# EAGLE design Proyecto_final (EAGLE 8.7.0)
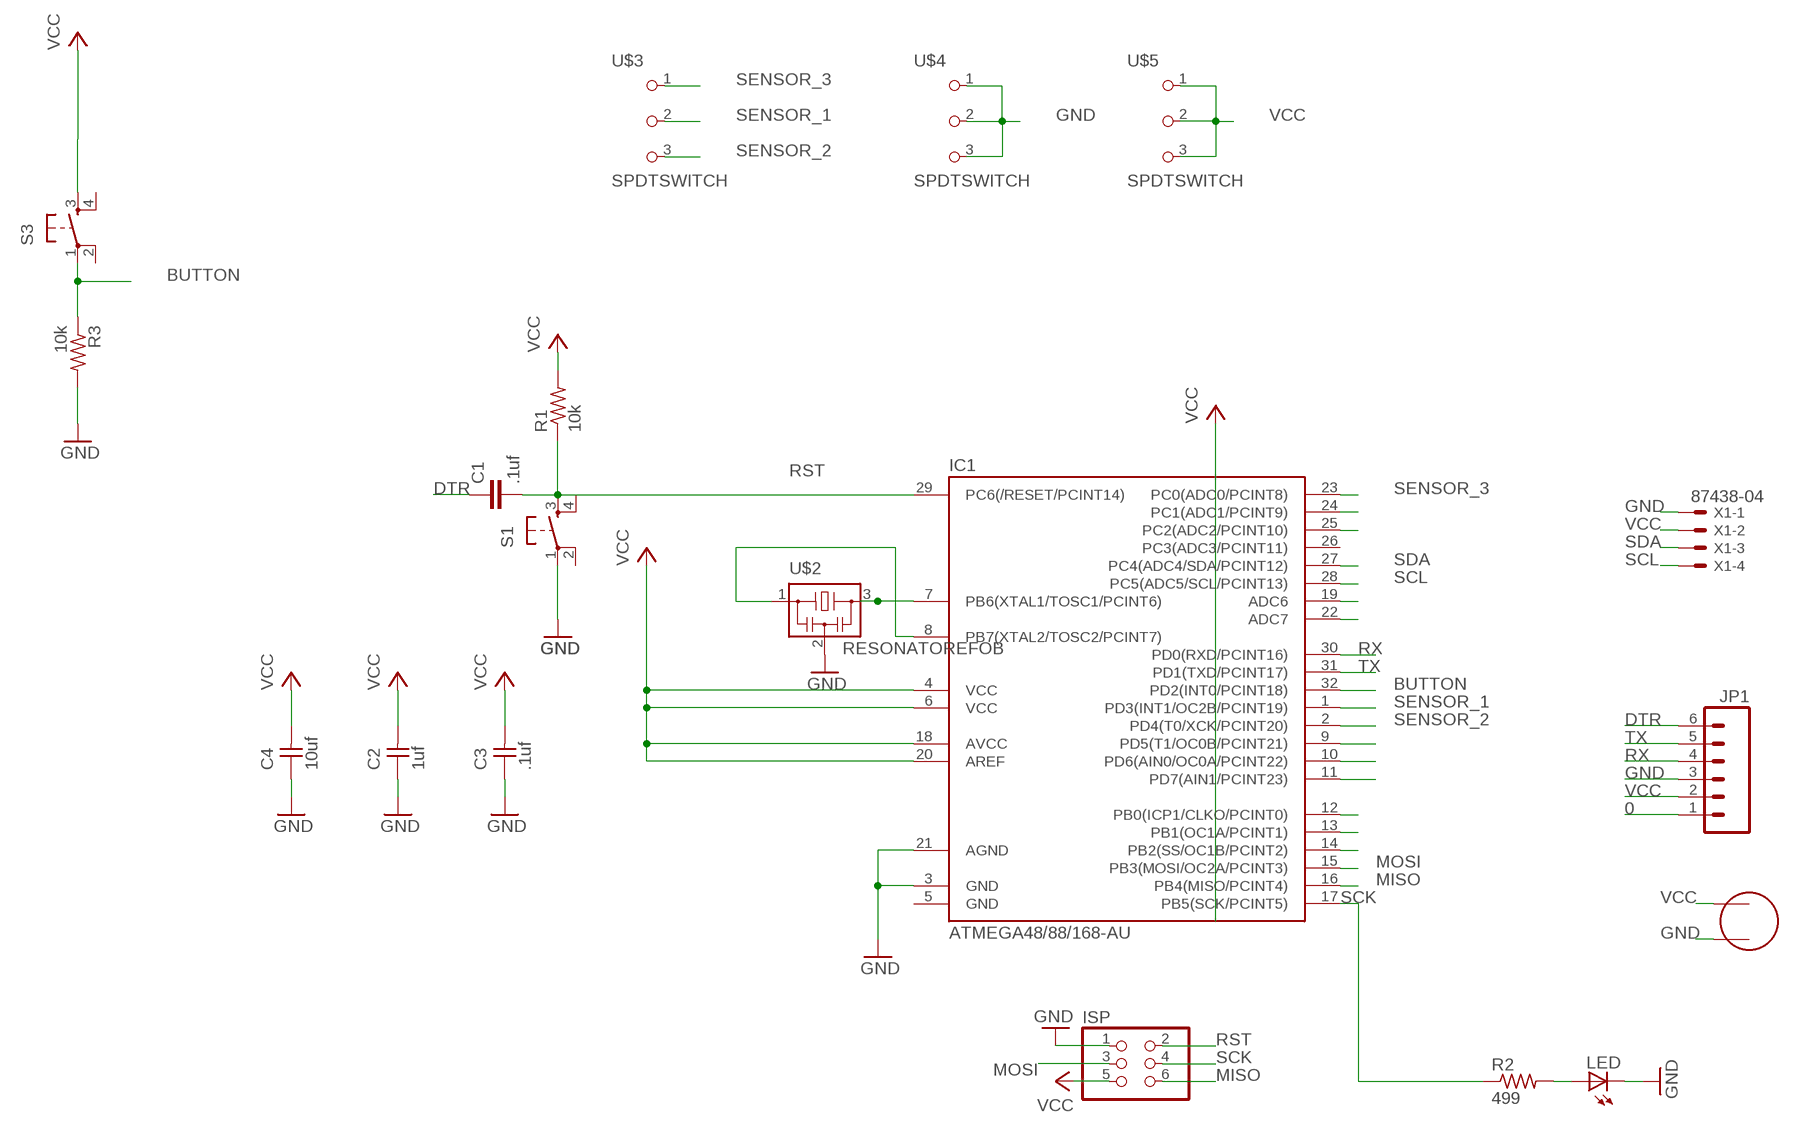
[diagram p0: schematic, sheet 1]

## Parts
C1  .1uf  C-EUC1206  [C1206]
C2  1uf  UNPOLARIZED_CAPACITOR1206  [1206]
C3  .1uf  UNPOLARIZED_CAPACITOR1206  [1206]
C4  10uf  UNPOLARIZED_CAPACITOR1206  [1206]
IC1  ATMEGA48/88/168-AU  [TQFP32-08]
ISP  PINHD-2X3-SMD  [2X03SMD]
JP1  M06SMD  [1X06-SMD]
LED  LED1206  [1206]
R1  10k  RESISTOR1206  [1206]
R2  499  RESISTOR1206  [1206]
R3  10k  RESISTOR1206  [1206]
S1  6MM_SWITCH6MM_SWITCH  [6MM_SWITCH]
S3  6MM_SWITCH6MM_SWITCH  [6MM_SWITCH]
U$1  ELECTRET  [ELECTRET_2742PBJ-A]
U$2  RESONATOREFOB  [EFOBM]
U$3  SPDTSWITCH  [SPDTSWITCH]
U$4  SPDTSWITCH  [SPDTSWITCH]
U$5  SPDTSWITCH  [SPDTSWITCH]
X1  87438-04  [87438-04]

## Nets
0: JP1.1
BUTTON: IC1.32(PD2(INT0/PCINT18)) R3.1 S3.1(P)
DTR: C1.1 JP1.6
GND: C2.1 C3.1 C4.1 IC1.3(GND) IC1.21(AGND) ISP.1 JP1.3 LED.2(C) R3.2 S1.1(P) U$1.P$2 U$2.2 U$4.1 U$4.2 U$4.3 X1.1
MISO: IC1.16(PB4(MISO/PCINT4)) ISP.6
MOSI: IC1.15(PB3(MOSI/OC2A/PCINT3)) ISP.3
N$1: IC1.8(PB7(XTAL2/TOSC2/PCINT7)) U$2.1
N$4: IC1.25(PC2(ADC2/PCINT10))
N$8: IC1.19(ADC6)
N$9: IC1.7(PB6(XTAL1/TOSC1/PCINT6)) U$2.3
N$10: IC1.22(ADC7)
N$14: IC1.9(PD5(T1/OC0B/PCINT21))
N$15: IC1.10(PD6(AIN0/OC0A/PCINT22))
N$16: IC1.11(PD7(AIN1/PCINT23))
N$17: IC1.14(PB2(SS/OC1B/PCINT2))
N$18: IC1.13(PB1(OC1A/PCINT1))
N$19: IC1.12(PB0(ICP1/CLKO/PCINT0))
N$23: LED.1(A) R2.2
RST: C1.2 IC1.29(PC6(/RESET/PCINT14)) ISP.2 R1.1 S1.3(S)
RST1: S3.3(S)
RX: IC1.30(PD0(RXD/PCINT16)) JP1.4
SCK: IC1.17(PB5(SCK/PCINT5)) ISP.4 R2.1
SCL: IC1.28(PC5(ADC5/SCL/PCINT13)) X1.4
SDA: IC1.27(PC4(ADC4/SDA/PCINT12)) X1.3
SENSOR_1: IC1.1(PD3(INT1/OC2B/PCINT19)) U$3.2
SENSOR_2: IC1.2(PD4(T0/XCK/PCINT20)) U$3.3
SENSOR_3: IC1.23(PC0(ADC0/PCINT8)) IC1.24(PC1(ADC1/PCINT9)) U$3.1
TX: IC1.31(PD1(TXD/PCINT17)) JP1.5
VCC: C2.2 C3.2 C4.2 IC1.4(VCC) IC1.6(VCC) IC1.18(AVCC) IC1.20(AREF) ISP.5 JP1.2 R1.2 U$1.P$1 U$5.1 U$5.2 U$5.3 X1.2
Unconnected: IC1.26(PC3(ADC3/PCINT11)) S1.2(P1) S1.4(S1) S3.2(P1) S3.4(S1)

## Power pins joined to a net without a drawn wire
GND: IC1.5(GND)

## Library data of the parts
C1 = rcl:C-EU: CAPACITOR, European symbol
C2-C4 = ng:UNPOLARIZED_CAPACITOR: unpolarized_capacitor
IC1 = atmega8:ATMEGA48/88/168
ISP = fab:PINHD-2X3-SMD: PIN HEADER
JP1 = SparkFun:M06: Header 6 Standard 6-pin 0.1" header. Use with straight break away headers (SKU : PRT-00116), right angle break away headers (PRT-00553), swiss pins (PRT-00743), machine pins (PRT-00117), and female headers (PRT-00115). Molex polarized connector foot print use with SKU : PRT-08094 with associated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
LED = ng:LED
R1-R3 = ng:RESISTOR
S1 S3 = ng:6MM_SWITCH: OMRON SWITCH
U$1 = fab:ELECTRET
U$2 = fab:RESONATOR
U$3-U$5 = fab:SPDTSWITCH
X1 = con-molex:87438-04: Wire-to-Board 1.50mm (.059") Pitch Header - Right Angle, SMT, Shrouded Source: http://www.molex.com/product/micro/87438.html; MF: MOLEX; OC_FARNELL: unknown; OC_NEWARK: unknown

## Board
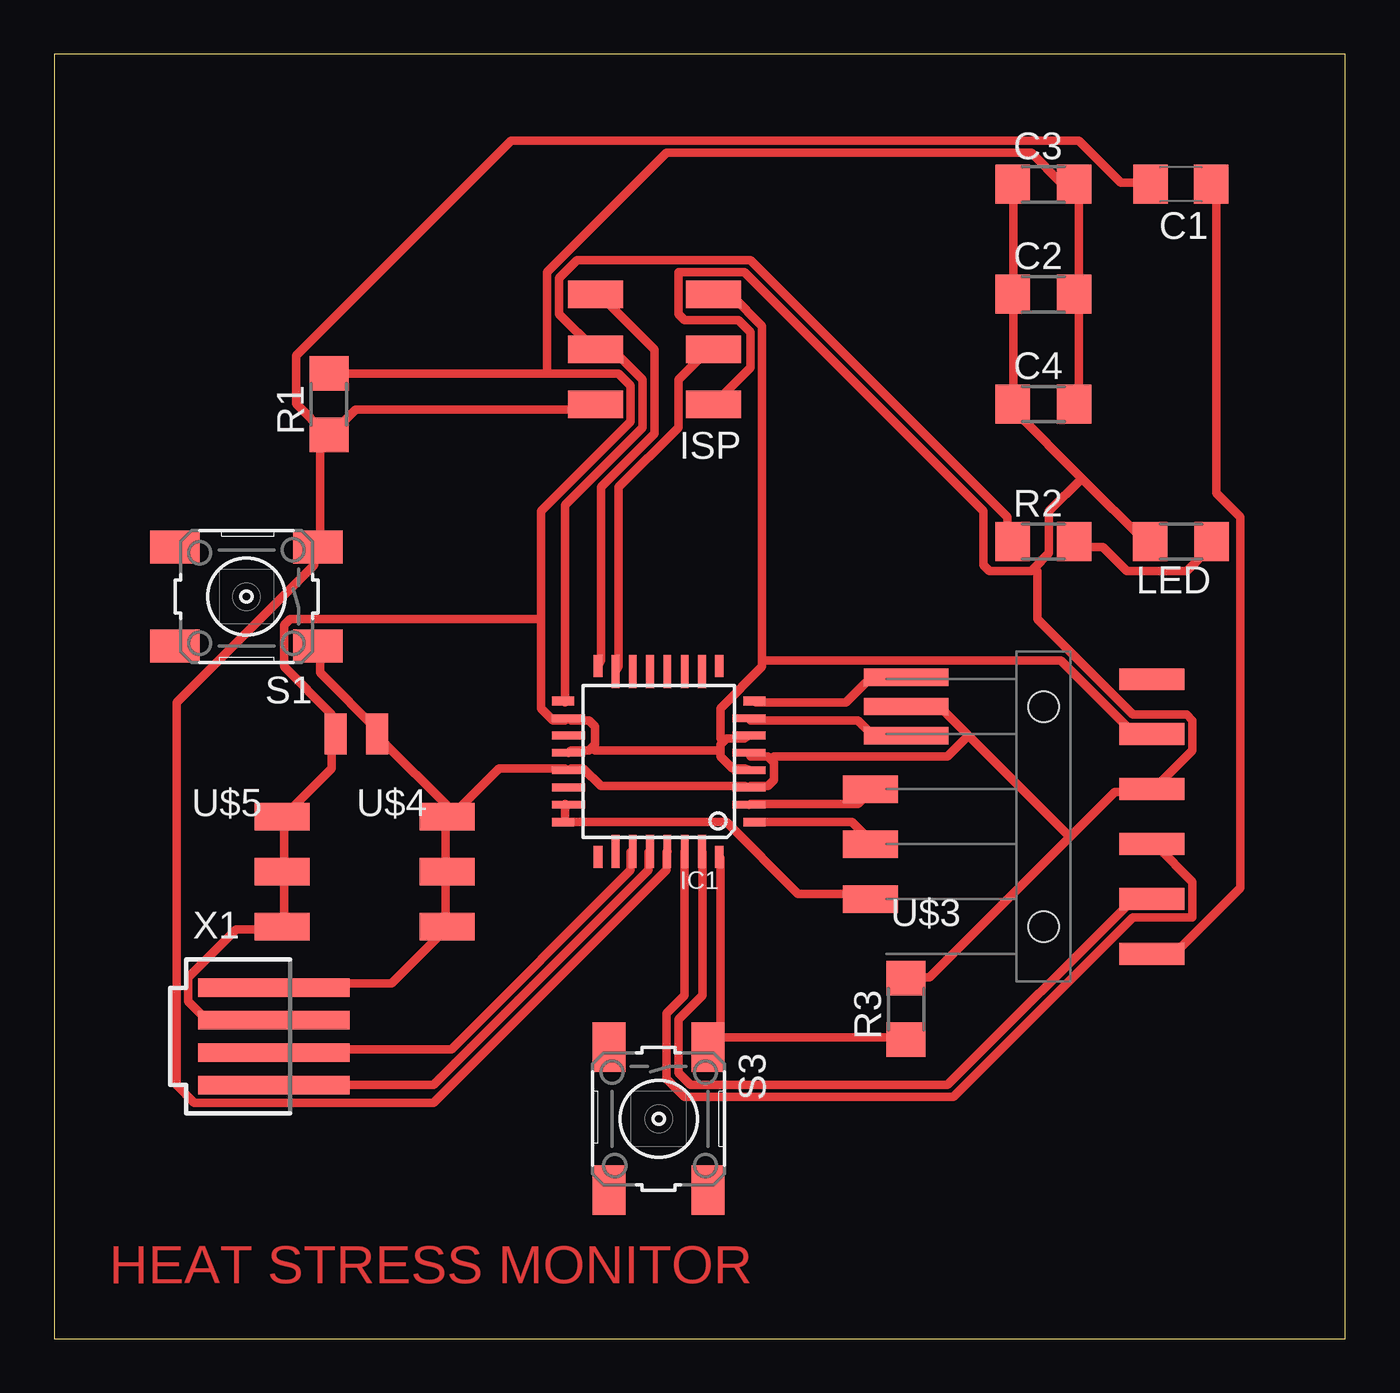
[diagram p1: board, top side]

Size 59.67 x 59.36 mm. Coordinates in mm from the lower left corner, seen from the top.
Outline: 0,0 59.67,0 59.67,59.36 0,59.36 0,0
Copper layers (1*16): Top 0.035mm / dielectric 1.5mm / Bottom 0.035mm
Design rules "default *": minimum track width 0.4mm, minimum drill 0.35mm, track to track 6mil, track to pad 6mil, pad to pad 6mil, via to via 6mil, smd to smd 6mil, copper to edge 40mil, drill to drill 6mil, minimum pad ring 10mil, minimum via ring 8mil, stop-mask expansion 4mil, vias tented up to drill 0mil, thermal gap 10mil

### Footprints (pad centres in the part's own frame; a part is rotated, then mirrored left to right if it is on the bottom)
C1206 = smd 1.6 x 1.8: 1 -1.4,0; 2 1.4,0
1206 = smd 1.6 x 1.803: 1 -1.422,0; 2 1.422,0
TQFP32-08 = smd 1.016 x 0.406: 1 -4.42,2.8; 8 -4.42,-2.8; 17 4.42,-2.8; 24 4.42,2.8 | smd 1.524 x 0.356: 2 -4.166,2; 3 -4.166,1.2; 4 -4.166,0.4; 5 -4.166,-0.4; 6 -4.166,-1.2; 7 -4.166,-2; 18 4.166,-2; 19 4.166,-1.2; 20 4.166,-0.4; 21 4.166,0.4; 22 4.166,1.2; 23 4.166,2 | smd 0.406 x 1.016: 9 -2.8,-4.42; 16 2.8,-4.42; 25 2.8,4.42; 32 -2.8,4.42 | smd 0.356 x 1.524: 10 -2,-4.166; 11 -1.2,-4.166; 12 -0.4,-4.166; 13 0.4,-4.166; 14 1.2,-4.166; 15 2,-4.166; 26 2,4.166; 27 1.2,4.166; 28 0.4,4.166; 29 -0.4,4.166; 30 -1.2,4.166; 31 -2,4.166
2X03SMD = smd 2.54 x 1.27: 1 -2.54,2.54; 2 2.92,2.54; 3 -2.54,0; 4 2.92,0; 5 -2.54,-2.54; 6 2.92,-2.54
1X06-SMD = smd 1 x 3: 1 -6.35,5; 2 -3.81,5; 3 -1.27,5; 4 1.27,5; 5 3.81,5; 6 6.35,5 | hole 1.4: -5.08,0; 5.08,0
6MM_SWITCH = smd 2.286 x 1.524: 1 -3.302,2.286; 2 3.302,2.286; 3 -3.302,-2.286; 4 3.302,-2.286
ELECTRET_2742PBJ-A = smd 1.016 x 1.905: P$1 -0.953,0; P$2 0.953,0
EFOBM = smd 0.8 x 3.9: 1 -1.35,0; 2 0,0; 3 1.35,0
SPDTSWITCH = smd 2.54 x 1.27: 1 0.38,2.54; 2 0.38,0; 3 0.38,-2.54
87438-04 = smd 7 x 0.85: 1 0,2.25; 2 0,0.75; 3 0,-0.75; 4 0,-2.25

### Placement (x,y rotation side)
C1  52.07,53.34 180 top
C2  45.72,48.26 0 top
C3  45.72,53.34 0 top
C4  45.72,43.18 0 top
IC1  27.94,26.67 180 top
ISP  27.94,45.72 180 top
JP1  45.72,24.13 270 top
LED  52.07,36.83 180 top
R1  12.7,43.18 90 top
R2  45.72,36.83 0 top
R3  39.37,15.24 90 top
S1  8.89,34.29 180 top
S3  27.94,10.16 270 top
U$1  13.97,27.94 0 top
U$2  39.37,29.21 270 top
U$3  38.1,22.86 180 top
U$4  17.78,21.59 0 top
U$5  10.16,21.59 0 top
X1  10.16,13.97 0 top

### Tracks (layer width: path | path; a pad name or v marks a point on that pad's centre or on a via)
BUTTON
  Top 0.4: IC1.32 30.79,22.22 30.79,14.21 30.23,13.66 S3.1 30.79,13.93 39.35,13.93 R3.1
DTR
  Top 0.4: C1.1 53.71,53.15 53.71,39.07 54.82,37.96 54.82,20.84 51.78,17.8 50.95,17.8 JP1.6
GND
  Top 0.4: 47.5,39.76 44.32,42.93 C4.1 44.32,43.21 44.32,48.18 C2.1 44.32,48.46 44.32,53.15 C3.1 | 47.5,39.76 50.4,36.86 LED.2 | 45.29,35.61 45.98,36.3 45.98,38.24 47.5,39.76 | 45.29,35.61 45.15,35.48 43.22,35.48 42.94,35.75 42.94,38.24 31.89,49.28 28.85,49.28 28.85,47.35 29.13,47.08 31.62,47.08 32.17,46.52 32.17,44.87 30.51,43.21 ISP.1 | 46.95,23.18 49.02,25.26 50.67,25.26 JP1.3 50.95,25.53 52.61,27.19 52.61,28.57 52.33,28.85 49.84,28.85 45.43,33.27 45.43,35.48 45.29,35.61 | 46.95,23.18 40.45,16.69 39.63,16.69 R3.2 | 46.95,23.18 42.25,27.88 | 42.25,27.88 41.01,29.12 39.63,29.12 U$2.2 | 33.14,26.77 33,26.91 32.17,26.91 IC1.5 | 33.14,26.77 33.27,26.64 33.27,25.81 33,25.53 32.17,25.53 IC1.3 31.89,25.53 25.26,25.53 24.44,26.36 23.88,26.36 IC1.21 23.61,26.36 20.57,26.36 18.36,24.15 U$4.1 | U$4.1 18.36,24.43 15.04,27.74 U$1.P$2 15.04,28.02 12.28,30.78 12.28,31.88 S1.1 | U$4.1 18.08,23.88 18.08,21.66 U$4.2 18.08,21.39 18.08,19.18 U$4.3 18.08,18.9 15.6,16.42 10.35,16.42 X1.1 | 42.25,27.88 41.28,26.91 33.27,26.91 33.14,26.77
MISO
  Top 0.4: IC1.16 25.26,31.33 25.26,39.34 27.75,41.83 27.75,45.69 25.26,48.18 ISP.6
MOSI
  Top 0.4: IC1.15 26.09,31.06 26.09,39.34 28.85,42.1 28.85,44.31 30.23,45.69 ISP.3
N$1
  Top 0.4: IC1.8 32.45,29.4 36.59,29.4 37.69,30.5 39.35,30.5 U$2.1
N$9
  Top 0.4: IC1.7 32.17,28.57 37.14,28.57 37.69,28.02 39.35,28.02 U$2.3
N$23
  Top 0.4: R2.2 47.36,36.58 48.46,36.58 49.57,35.48 52.33,35.48 53.44,36.58 LED.1
RST
  Top 0.4: IC1.29 28.3,22.49 28.3,21.66 17.53,10.89 6.48,10.89 5.65,11.72 5.65,29.4 12.01,35.75 12.01,36.3 S1.3 12.28,36.58 12.28,41.83 R1.1 | C1.2 50.4,53.43 49.29,53.43 47.36,55.36 21.12,55.36 11.18,45.42 11.18,43.21 12.56,41.83 R1.1 | ISP.2 24.99,42.93 13.94,42.93 12.83,41.83 R1.1
RX
  Top 0.4: IC1.30 29.13,15.86 28.3,15.04 28.3,12 29.13,11.17 41.56,11.17 49.84,19.45 52.61,19.45 52.61,21.11 50.95,22.77 JP1.4
SCK
  Top 0.4: IC1.17 23.61,29.4 23.61,38.51 27.2,42.1 27.2,44.31 25.82,45.69 25.26,45.69 ISP.4 24.99,45.69 23.33,47.35 23.33,49.01 24.16,49.84 32.17,49.84 44.05,37.96 44.05,36.86 R2.1
SCL
  Top 0.4: IC1.28 27.47,22.49 27.47,21.66 17.53,11.72 10.35,11.72 X1.4
SDA
  Top 0.4: IC1.27 26.64,22.49 26.64,21.66 18.36,13.38 10.35,13.38 X1.3
SENSOR_1
  Top 0.4: IC1.1 32.45,23.88 36.86,23.88 37.69,23.05 U$3.2
SENSOR_2
  Top 0.4: IC1.2 32.17,24.7 37.14,24.7 37.69,25.26 U$3.3
SENSOR_3
  Top 0.4: 23.61,23.88 23.61,24.7 IC1.23 | 23.61,23.88 31.06,23.88 34.38,20.56 37.69,20.56 U$3.1 | 23.61,23.88 IC1.24
TX
  Top 0.4: IC1.31 29.96,22.49 29.96,15.86 28.85,14.76 28.85,12.27 29.41,11.72 41.28,11.72 49.84,20.28 50.67,20.28 JP1.5
VCC
  Top 0.4: X1.2 10.07,14.76 7.03,14.76 6.21,15.59 6.21,16.69 8.41,18.9 10.35,18.9 U$5.3 10.62,19.18 10.62,21.39 U$5.2 10.62,21.66 10.62,23.88 U$5.1 10.62,24.15 12.83,26.36 12.83,27.74 U$1.P$1 12.83,28.02 12.83,28.85 10.62,31.06 10.62,32.99 10.9,33.27 22.5,33.27 | C4.2 47.36,43.21 47.36,48.18 C2.2 47.36,48.46 47.36,53.15 C3.2 47.08,53.43 46.53,53.43 45.15,54.81 28.3,54.81 22.78,49.28 22.78,44.59 | 30.79,27.19 30.79,27.46 30.92,27.6 | 30.79,27.19 30.79,26.91 31.34,26.36 31.89,26.36 IC1.4 | 30.92,27.6 31.06,27.74 31.89,27.74 IC1.6 | 24.85,27.33 24.99,27.46 24.99,28.29 24.71,28.57 23.88,28.57 IC1.18 23.61,28.57 23.05,28.57 22.5,29.12 22.5,33.27 | 24.85,27.33 24.71,27.19 23.88,27.19 IC1.20 | 22.78,44.59 26.09,44.59 26.64,44.04 26.64,42.38 22.5,38.24 22.5,33.27 | 22.78,44.59 12.83,44.59 R1.2 | 30.79,27.19 24.99,27.19 24.85,27.33 | 32.72,31.33 32.72,31.06 30.79,29.12 30.79,27.74 30.92,27.6 | 32.72,31.33 32.72,46.8 31.34,48.18 30.51,48.18 ISP.5 | 32.72,31.33 46.53,31.33 49.84,28.02 50.67,28.02 JP1.2

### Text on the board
Top: HEAT STRESS MONITOR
